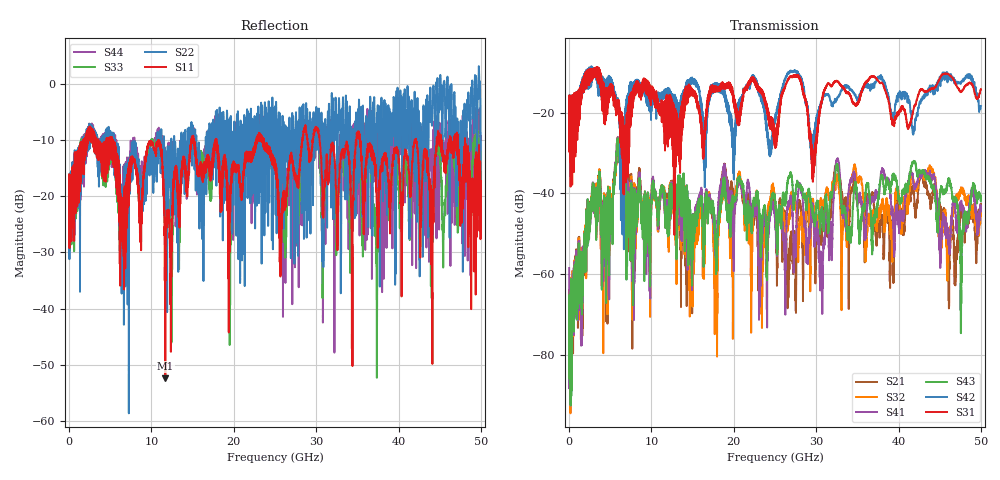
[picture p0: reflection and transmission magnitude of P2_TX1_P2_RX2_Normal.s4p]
!Keysight Technologies,N5225B,MY57041031,A.13.20.10
!Date: Friday, May 31, 2019 11:28:59
!Correction: S11(Full 4 Port(1,2,3,4))
!S12(Full 4 Port(1,2,3,4))
!S13(Full 4 Port(1,2,3,4))
!S14(Full 4 Port(1,2,3,4))
!S21(Full 4 Port(1,2,3,4))
!S22(Full 4 Port(1,2,3,4))
!S23(Full 4 Port(1,2,3,4))
!S24(Full 4 Port(1,2,3,4))
!S31(Full 4 Port(1,2,3,4))
!S32(Full 4 Port(1,2,3,4))
!S33(Full 4 Port(1,2,3,4))
!S34(Full 4 Port(1,2,3,4))
!S41(Full 4 Port(1,2,3,4))
!S42(Full 4 Port(1,2,3,4))
!S43(Full 4 Port(1,2,3,4))
!S44(Full 4 Port(1,2,3,4))
!S4P File: Measurements: <S11,S12,S13,S14>,
!<S21,S22,S23,S24>,
!<S31,S32,S33,S34>,
!<S41,S42,S43,S44>:
# Hz S  dB  R 50.0
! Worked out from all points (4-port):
!   5000 points, 10 MHz to 50 GHz, reference 50 ohm
!   strongest paths, dB at 10 MHz, 12.51 GHz, 25.01 GHz, 37.51 GHz, 50 GHz:
!     S31: -19.5, -17.3, -28.7, -12.1, -14.2
!     S42: -19.5, -15.6, -21.7, -11.1, -18.4
!     S43: -79.6, -40.4, -41.3, -41.3, -41.2
!     S41: -58.4, -38.0, -45.6, -40.8, -43.6
!     S32: -64.1, -39.8, -41.9, -45.3, -45.1
!     S21: -63.9, -37.6, -45.4, -47.8, -42.7
!   lowest |S11| = -52.4 dB at 11.69 GHz (marker M1), VSWR 1.00, Z = 49.8 - j0.175 ohm
!   |S11| at or under -10 dB: 5.36 GHz to 10.81 GHz (5.449 GHz wide, 67.4 % of centre); 17.89 GHz to 22.7 GHz (4.804 GHz wide, 23.7 % of centre); 35.31 GHz to 41.96 GHz (6.647 GHz wide, 17.2 % of centre)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
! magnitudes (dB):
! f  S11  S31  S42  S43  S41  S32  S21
! 10 MHz  -19.6  -19.5  -19.5  -79.6  -58.4  -64.1  -63.9
! 6 GHz  -15.2  -17.7  -18.8  -26.6  -26.3  -26.5  -26.3
! 11.69 GHz  -52.4  -23.1  -16.1  -43.6  -43.4  -42.3  -42.3
! 14.98 GHz  -9.2  -15.4  -12.0  -47.4  -47.5  -51.4  -49.6
! 27.75 GHz  -17.8  -10.7  -10.0  -37.2  -41.0  -50.7  -46.9
! 29.65 GHz  -9.5  -36.0  -26.7  -45.5  -45.0  -42.3  -43.3
! 50 GHz  -17.3  -14.2  -18.4  -41.2  -43.6  -45.1  -42.7
